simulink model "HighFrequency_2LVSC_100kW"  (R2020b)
settings: Solver=ode45  StartTime=0.0  StopTime=360  RelTol=1e-4  EnableMultiTasking=on
undefined symbols (not defined in the file): A, A_extheat, A_mp, AceH, AceL, ad0H, ad0L, ad1H, ad1L, ad2H, ad2L, AfH, AfL, at0H, at0L, at1H, at1L, at2H, at2L, C_V_ref, Cha1, CjcD, CjcT, Converters, Cp_Cu, Cp_wall, filter, FILTER_INT, fs, Grid_V, IGBT_len, IGBT_wid, Iq_init, J, k_box, k_mp, k_tp, kI_speed, kP_speed, L_equi, L_f1, Len_mp, Ls, nSpp, omega_m_init, omega_s, p, phi_pm, R1_cauer, R1D_bp, R2_cauer, R_f1, R_jc1, R_jc2, R_jc3, R_jc4, R_wall, Radius, RceH, RceL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
libraries: simulink x5, powerlib_meascontrol x2, pid_lib x2, cstblocks x1
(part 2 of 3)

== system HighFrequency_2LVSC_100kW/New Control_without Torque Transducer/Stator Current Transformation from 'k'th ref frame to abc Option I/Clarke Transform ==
  in_1 : Inport
  in_2 : Inport  Port=2
  1/w2 : Constant  Value=1/sqrt(2)
  1/w6 : Constant  Value=1/sqrt(6)
  Product : Product  InputSameDT=on  RndMeth=Zero  SaturateOnIntegerOverflow=on
  Product1 : Product  InputSameDT=on  RndMeth=Zero  SaturateOnIntegerOverflow=on
  Product2 : Product  InputSameDT=on  RndMeth=Zero  SaturateOnIntegerOverflow=on
  Sum : Sum  Inputs=-+  InputSameDT=on  SaturateOnIntegerOverflow=on
  Sum1 : Sum  Inputs=--  InputSameDT=on  SaturateOnIntegerOverflow=on
  w2/w3 : Constant  Value=sqrt(2/3)
  out_1 : Outport  VectorParamsAs1DForOutWhenUnconnected=off
  out_2 : Outport  Port=2  VectorParamsAs1DForOutWhenUnconnected=off
  out_3 : Outport  Port=3  VectorParamsAs1DForOutWhenUnconnected=off
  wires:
  in_1/1 -> Product/2, Product1/1
  Product2/1 -> Sum1/2, Sum/2
  Product1/1 -> Sum1/1, Sum/1
  1/w2/1 -> Product2/2
  1/w6/1 -> Product1/2
  w2/w3/1 -> Product/1
  Product/1 -> out_1/1
  Sum/1 -> out_2/1
  in_2/1 -> Product2/1
  Sum1/1 -> out_3/1

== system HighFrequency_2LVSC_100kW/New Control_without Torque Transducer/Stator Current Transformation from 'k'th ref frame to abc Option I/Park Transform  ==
  in_1 : Inport
  in_2 : Inport  Port=2
  in_3 : Inport  Port=3
  Product{,1..3} (4 alike) : Product  InputSameDT=on  RndMeth=Zero  SaturateOnIntegerOverflow=on
  Sum : Sum  Inputs=+-  InputSameDT=on  SaturateOnIntegerOverflow=on
  Sum1 : Sum  InputSameDT=on  SaturateOnIntegerOverflow=on
  cos : Fcn  Expr=cos(u(1))
  sin : Fcn  Expr=sin(u(1))
  out_1 : Outport  VectorParamsAs1DForOutWhenUnconnected=off
  out_2 : Outport  Port=2  VectorParamsAs1DForOutWhenUnconnected=off
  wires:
  Product2/1 -> Sum/2
  Product3/1 -> Sum1/1
  Product1/1 -> Sum/1
  Product/1 -> Sum1/2
  in_3/1 -> sin/1, cos/1
  sin/1 -> Product3/2, Product2/2
  cos/1 -> Product/2, Product1/2
  Sum/1 -> out_1/1
  Sum1/1 -> out_2/1
  in_1/1 -> Product3/1, Product1/1
  in_2/1 -> Product/1, Product2/1

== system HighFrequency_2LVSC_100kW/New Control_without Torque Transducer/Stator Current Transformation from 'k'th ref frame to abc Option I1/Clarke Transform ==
  in_1 : Inport
  in_2 : Inport  Port=2
  1/w2 : Constant  Value=1/sqrt(2)
  1/w6 : Constant  Value=1/sqrt(6)
  Product : Product  InputSameDT=on  RndMeth=Zero  SaturateOnIntegerOverflow=on
  Product1 : Product  InputSameDT=on  RndMeth=Zero  SaturateOnIntegerOverflow=on
  Product2 : Product  InputSameDT=on  RndMeth=Zero  SaturateOnIntegerOverflow=on
  Sum : Sum  Inputs=-+  InputSameDT=on  SaturateOnIntegerOverflow=on
  Sum1 : Sum  Inputs=--  InputSameDT=on  SaturateOnIntegerOverflow=on
  w2/w3 : Constant  Value=sqrt(2/3)
  out_1 : Outport  VectorParamsAs1DForOutWhenUnconnected=off
  out_2 : Outport  Port=2  VectorParamsAs1DForOutWhenUnconnected=off
  out_3 : Outport  Port=3  VectorParamsAs1DForOutWhenUnconnected=off
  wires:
  Sum1/1 -> out_3/1
  in_2/1 -> Product2/1
  Sum/1 -> out_2/1
  Product/1 -> out_1/1
  w2/w3/1 -> Product/1
  1/w6/1 -> Product1/2
  1/w2/1 -> Product2/2
  Product1/1 -> Sum/1, Sum1/1
  Product2/1 -> Sum/2, Sum1/2
  in_1/1 -> Product1/1, Product/2

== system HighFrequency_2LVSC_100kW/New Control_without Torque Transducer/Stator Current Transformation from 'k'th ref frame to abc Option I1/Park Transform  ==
  in_1 : Inport
  in_2 : Inport  Port=2
  in_3 : Inport  Port=3
  Product{,1..3} (4 alike) : Product  InputSameDT=on  RndMeth=Zero  SaturateOnIntegerOverflow=on
  Sum : Sum  Inputs=+-  InputSameDT=on  SaturateOnIntegerOverflow=on
  Sum1 : Sum  InputSameDT=on  SaturateOnIntegerOverflow=on
  cos : Fcn  Expr=cos(u(1))
  sin : Fcn  Expr=sin(u(1))
  out_1 : Outport  VectorParamsAs1DForOutWhenUnconnected=off
  out_2 : Outport  Port=2  VectorParamsAs1DForOutWhenUnconnected=off
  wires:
  in_2/1 -> Product2/1, Product/1
  in_1/1 -> Product1/1, Product3/1
  Sum1/1 -> out_2/1
  Sum/1 -> out_1/1
  cos/1 -> Product1/2, Product/2
  sin/1 -> Product2/2, Product3/2
  in_3/1 -> cos/1, sin/1
  Product/1 -> Sum1/2
  Product1/1 -> Sum/1
  Product3/1 -> Sum1/1
  Product2/1 -> Sum/2

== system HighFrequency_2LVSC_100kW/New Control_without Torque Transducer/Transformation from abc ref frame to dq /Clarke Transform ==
  note: u_b
  note: u_c
  note: u_a
  note: u_alpha
  note: u_beta
  in_1 : Inport
  in_2 : Inport  Port=2
  in_3 : Inport  Port=3
  1/w2 : Constant  Value=1/sqrt(2)
  1/w6 : Constant  Value=1/sqrt(6)
  Product{,1..3} (4 alike) : Product  InputSameDT=on  RndMeth=Zero  SaturateOnIntegerOverflow=on
  Sum : Sum  Inputs=+--  InputSameDT=on  SaturateOnIntegerOverflow=on
  Sum1 : Sum  Inputs=+-  InputSameDT=on  SaturateOnIntegerOverflow=on
  w2/w3 : Constant  Value=sqrt(2/3)
  out_1 : Outport  VectorParamsAs1DForOutWhenUnconnected=off
  out_2 : Outport  Port=2  VectorParamsAs1DForOutWhenUnconnected=off
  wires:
  Product3/1 -> out_2/1
  Sum/1 -> out_1/1
  in_1/1 -> Product/2
  Product/1 -> Sum/1
  w2/w3/1 -> Product/1
  1/w6/1 -> Product1/2, Product2/2
  Product1/1 -> Sum/2
  in_2/1 -> Sum1/1, Product1/1
  in_3/1 -> Sum1/2, Product2/1
  Sum1/1 -> Product3/1
  Product2/1 -> Sum/3
  1/w2/1 -> Product3/2

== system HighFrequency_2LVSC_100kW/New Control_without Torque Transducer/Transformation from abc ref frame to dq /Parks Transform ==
  in_1 : Inport
  in_2 : Inport  Port=2
  in_3 : Inport  Port=3
  Product{,1..3} (4 alike) : Product  InputSameDT=on  RndMeth=Zero  SaturateOnIntegerOverflow=on
  Sum : Sum  Inputs=+-  InputSameDT=on  SaturateOnIntegerOverflow=on
  Sum1 : Sum  InputSameDT=on  SaturateOnIntegerOverflow=on
  cos : Fcn  Expr=cos(u(1))
  sin : Fcn  Expr=sin(u(1))
  out_1 : Outport  VectorParamsAs1DForOutWhenUnconnected=off
  out_2 : Outport  Port=2  VectorParamsAs1DForOutWhenUnconnected=off
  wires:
  Product2/1 -> Sum/2
  Product3/1 -> Sum1/1
  Product1/1 -> Sum/1
  Product/1 -> Sum1/2
  in_3/1 -> sin/1, cos/1
  sin/1 -> Product3/2, Product2/2
  cos/1 -> Product/2, Product1/2
  Sum/1 -> out_1/1
  Sum1/1 -> out_2/1
  in_1/1 -> Product3/1, Product1/1
  in_2/1 -> Product/1, Product2/1

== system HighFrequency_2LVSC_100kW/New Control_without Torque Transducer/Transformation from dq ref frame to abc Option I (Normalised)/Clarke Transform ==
  in_1 : Inport
  in_2 : Inport  Port=2
  1/w2 : Constant  Value=1/sqrt(2)
  1/w6 : Constant  Value=1/sqrt(6)
  Product : Product  InputSameDT=on  RndMeth=Zero  SaturateOnIntegerOverflow=on
  Product1 : Product  InputSameDT=on  RndMeth=Zero  SaturateOnIntegerOverflow=on
  Product2 : Product  InputSameDT=on  RndMeth=Zero  SaturateOnIntegerOverflow=on
  Sum : Sum  Inputs=-+  InputSameDT=on  SaturateOnIntegerOverflow=on
  Sum1 : Sum  Inputs=--  InputSameDT=on  SaturateOnIntegerOverflow=on
  w2/w3 : Constant  Value=sqrt(2/3)
  out_1 : Outport  VectorParamsAs1DForOutWhenUnconnected=off
  out_2 : Outport  Port=2  VectorParamsAs1DForOutWhenUnconnected=off
  out_3 : Outport  Port=3  VectorParamsAs1DForOutWhenUnconnected=off
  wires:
  in_1/1 -> Product/2, Product1/1
  Product2/1 -> Sum1/2, Sum/2
  Product1/1 -> Sum1/1, Sum/1
  1/w2/1 -> Product2/2
  1/w6/1 -> Product1/2
  w2/w3/1 -> Product/1
  Product/1 -> out_1/1
  Sum/1 -> out_2/1
  in_2/1 -> Product2/1
  Sum1/1 -> out_3/1

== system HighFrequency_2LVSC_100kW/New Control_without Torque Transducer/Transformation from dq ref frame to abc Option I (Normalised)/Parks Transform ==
  in_1 : Inport
  in_2 : Inport  Port=2
  in_3 : Inport  Port=3
  Product{,1..3} (4 alike) : Product  InputSameDT=on  RndMeth=Zero  SaturateOnIntegerOverflow=on
  Sum : Sum  Inputs=+-  InputSameDT=on  SaturateOnIntegerOverflow=on
  Sum1 : Sum  InputSameDT=on  SaturateOnIntegerOverflow=on
  cos : Fcn  Expr=cos(u(1))
  sin : Fcn  Expr=sin(u(1))
  out_1 : Outport  VectorParamsAs1DForOutWhenUnconnected=off
  out_2 : Outport  Port=2  VectorParamsAs1DForOutWhenUnconnected=off
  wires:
  Product2/1 -> Sum/2
  Product3/1 -> Sum1/1
  Product1/1 -> Sum/1
  Product/1 -> Sum1/2
  in_3/1 -> sin/1, cos/1
  sin/1 -> Product3/2, Product2/2
  cos/1 -> Product/2, Product1/2
  Sum/1 -> out_1/1
  Sum1/1 -> out_2/1
  in_1/1 -> Product3/1, Product1/1
  in_2/1 -> Product/1, Product2/1

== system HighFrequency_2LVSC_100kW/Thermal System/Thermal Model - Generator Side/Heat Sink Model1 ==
  PT1/D1 : Inport
  Flow Rate : Inport  Port=2
  MATLAB Function : MATLAB Function  TreatAsAtomicUnit=on
  Thermal Capacitance : Constant  Value=5.8824e+03
  "Thermal System " : Subsystem
  Tha1 : Outport  VectorParamsAs1DForOutWhenUnconnected=off
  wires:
  "Thermal System "/1(Tha) -> Tha1/1
  MATLAB Function/1(y) -> "Thermal System "/2(1/R_th)  "1/R_th"
  Flow Rate/1 -> MATLAB Function/1(u)
  PT1/D1/1 -> "Thermal System "/1(P1/D1)
  Thermal Capacitance/1 -> "Thermal System "/3(C)

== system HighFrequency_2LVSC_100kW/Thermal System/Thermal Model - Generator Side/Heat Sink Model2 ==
  PT1/D1 : Inport
  Flow Rate : Inport  Port=2
  1/Rha1 : Constant  Value=1/Rha1
  MATLAB Function : MATLAB Function  Commented=on  TreatAsAtomicUnit=on
  Thermal Capacitance : Constant  Commented=on  Value=5.8824e+03
  Thermal Capacitance1 : Constant  Value=Cha1
  "Thermal System " : Subsystem
  Tha1 : Outport  VectorParamsAs1DForOutWhenUnconnected=off
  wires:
  "Thermal System "/1(Tha) -> Tha1/1
  Flow Rate/1 -> MATLAB Function/1(u)
  PT1/D1/1 -> "Thermal System "/1(P1/D1)
  Thermal Capacitance1/1 -> "Thermal System "/3(C)
  1/Rha1/1 -> "Thermal System "/2(1/R_th)

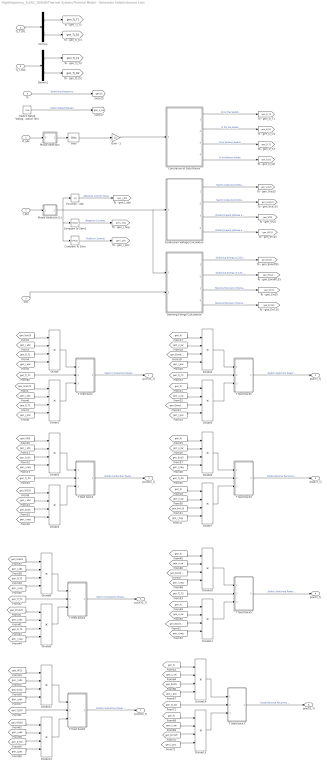
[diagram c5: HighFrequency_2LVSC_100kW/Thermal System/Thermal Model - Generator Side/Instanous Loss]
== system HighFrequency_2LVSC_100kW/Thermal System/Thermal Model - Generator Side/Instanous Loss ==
  D_abc : Inport
  I_abc : Inport  Port=2
  Vdc : Inport  Port=3
  fs : Inport  Port=4
  Tj_T1D1 : Inport  Port=5
  Tj_T2D2 : Inport  Port=6
  Bias : Bias  Bias=1
  Calculation of Duty Ratios : Subsystem
  Compare To Zero : simulink/Logic and Bit Operations/Compare To Zero  relop=>=  OutDataTypeStr=boolean
  Compare To Zero1 : simulink/Logic and Bit Operations/Compare To Zero  relop=<  OutDataTypeStr=boolean
  Conduction Voltage Calculation : Subsystem
  Demux : Demux  Outputs=2
  Demux1 : Demux  Outputs=2
  Divide{,1..15} (16 alike) : Product  Inputs=****
  Function - abs : Abs
  Gain - 1 : Gain  Gain=1/2
  Phase Selection : Subsystem
  Phase Selection (1) : Subsystem
  Switch Rated Voltage (from Initialisation file) : Constant  Value=Usw
  Swithing Energy Calculation : Subsystem
  T feed back : Subsystem
  T feed back1 : Subsystem
  T feed back2 : Subsystem
  T feed back3 : Subsystem
  T feed back4 : Subsystem
  T feed back5 : Subsystem
  T feed back6 : Subsystem
  T feed back7 : Subsystem
  pconT1_Tj : Outport  VectorParamsAs1DForOutWhenUnconnected=off
  pswT1_Tj : Outport  Port=2  VectorParamsAs1DForOutWhenUnconnected=off
  pconD1_Tj : Outport  Port=3  VectorParamsAs1DForOutWhenUnconnected=off
  pswD1_Tj : Outport  Port=4  VectorParamsAs1DForOutWhenUnconnected=off
  pconT2_Tj : Outport  Port=5  VectorParamsAs1DForOutWhenUnconnected=off
  pswT2_Tj : Outport  Port=6  VectorParamsAs1DForOutWhenUnconnected=off
  pconD2_Tj : Outport  Port=7  VectorParamsAs1DForOutWhenUnconnected=off
  pswD2_Tj : Outport  Port=8  VectorParamsAs1DForOutWhenUnconnected=off
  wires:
  D_abc/1 -> Phase Selection/1(In)
  Calculation of Duty Ratios/1(D_T1) -> [gen_D_T1]  "D for Top Switch"
  Calculation of Duty Ratios/2(D_D1) -> [gen_D_D1]  "D for Top Diode"
  Calculation of Duty Ratios/3(D_T2) -> [gen_D_T2]  "D for Bottom Switch"
  Calculation of Duty Ratios/4(D_D2) -> [gen_D_D2]  "D for Bottom Diode"
  Conduction Voltage Calculation/2(Vce 125) -> [gen_Vce125]  "Switch Collector-Emitter Voltage at 125degC"
  Conduction Voltage Calculation/4(Vf 125) -> [gen_Vf125]  "Diode Forward Voltage at 125degC"
  Conduction Voltage Calculation/1(Vce 25) -> [gen_Vce25]  "Switch Collector-Emitter Voltage at 25degC"
  Conduction Voltage Calculation/3(Vf 25) -> [gen_Vf25]  "Diode Forward Voltage at 25degC"
  Swithing Energy Calculation/4(Err 125) -> [gen_Err125]  "Reverse Recovery Energy at 125degC"
  Swithing Energy Calculation/2(Esw 125) -> [gen_Eonoff125]  "Switching Energy at 125degC"
  Swithing Energy Calculation/3(Err 25) -> [gen_Err25]  "Reverse Recovery Energy at 25degC"
  Swithing Energy Calculation/1(Esw 25) -> [gen_Eonoff25]  "Switching Energy at 25degC"
  Compare To Zero1/1 -> [gen_i_neg]  "Negative Currents"
  Compare To Zero/1 -> [gen_i_pos]  "Positive Currents"
  fs/1 -> [gen_fs]  "Switching Frequency"
  [gen_i_abs] -> Divide/2
  [gen_D_T1] -> Divide/3
  [gen_i_pos] -> Divide/4
  Function - abs/1 -> [gen_i_abs]  "Absolute Current Value"
  [gen_Vce125] -> Divide1/1
  [gen_i_abs] -> Divide1/2
  [gen_D_T1] -> Divide1/3
  [gen_i_pos] -> Divide1/4
  [gen_Vce25] -> Divide/1
  [gen_i_abs] -> Divide2/2
  [gen_D_D1] -> Divide2/3
  [gen_i_neg] -> Divide2/4
  [gen_Vf125] -> Divide3/1
  [gen_i_abs] -> Divide3/2
  [gen_D_D1] -> Divide3/3
  [gen_i_neg] -> Divide3/4
  [gen_Vf25] -> Divide2/1
  [gen_fs] -> Divide4/1
  [gen_u_sw] -> Divide4/2
  Switch Rated Voltage (from Initialisation file)/1 -> [gen_u_sw]  "Switch Rated Voltage"
  [gen_Eonoff25] -> Divide4/3
  [gen_i_pos] -> Divide4/4
  [gen_fs] -> Divide5/1
  [gen_u_sw] -> Divide5/2
  [gen_Eonoff125] -> Divide5/3
  [gen_i_pos] -> Divide5/4
  [gen_fs] -> Divide6/1
  [gen_u_sw] -> Divide6/2
  [gen_Err25] -> Divide6/3
  [gen_i_neg] -> Divide6/4
  [gen_fs] -> Divide7/1
  [gen_u_sw] -> Divide7/2
  [gen_Err125] -> Divide7/3
  [gen_i_neg] -> Divide7/4
  Divide4/1 -> T feed back1/1(TL)
  Divide5/1 -> T feed back1/3(TH)
  Divide/1 -> T feed back/1(TL)
  Divide1/1 -> T feed back/3(TH)
  T feed back/1(p_Tj) -> pconT1_Tj/1  "Switch Conduction Power Loss at Tj"
  Tj_T1D1/1 -> Demux/1
  Demux/1 -> [gen_Tj_T1]
  Demux/2 -> [gen_Tj_D1]
  [gen_Tj_T1] -> T feed back/2(Tj)
  [gen_Tj_T1] -> T feed back1/2(Tj)
  T feed back1/1(p_Tj) -> pswT1_Tj/1  "Switch Switching Power Loss at Tj"
  Divide2/1 -> T feed back2/1(TL)
  Divide3/1 -> T feed back2/3(TH)
  [gen_Tj_D1] -> T feed back2/2(Tj)
  T feed back2/1(p_Tj) -> pconD1_Tj/1  "Diode Conduction Power Loss at Tj"
  [gen_Tj_D1] -> T feed back3/2(Tj)
  Divide6/1 -> T feed back3/1(TL)
  Divide7/1 -> T feed back3/3(TH)
  T feed back3/1(p_Tj) -> pswD1_Tj/1  "Diode Reverse Recovery Power Loss at Tj"
  I_abc/1 -> Phase Selection (1)/1(In)
  Vdc/1 -> Swithing Energy Calculation/2(Vdc)
  Phase Selection (1)/1(Out) -> Swithing Energy Calculation/1(i_abc), Conduction Voltage Calculation/1(i_abc), Compare To Zero/1, Compare To Zero1/1, Function - abs/1
  Bias/1 -> Gain - 1/1
  Phase Selection/1(Out) -> Bias/1
  Gain - 1/1 -> Calculation of Duty Ratios/1(Dabc)
  Tj_T2D2/1 -> Demux1/1
  Demux1/1 -> [gen_Tj_T2]
  Demux1/2 -> [gen_Tj_D2]
  [gen_i_abs] -> Divide8/2
  [gen_D_T2] -> Divide8/3
  [gen_i_neg] -> Divide8/4
  [gen_Vce125] -> Divide9/1
  [gen_i_abs] -> Divide9/2
  [gen_D_T2] -> Divide9/3
  [gen_i_neg] -> Divide9/4
  [gen_Vce25] -> Divide8/1
  Divide8/1 -> T feed back4/1(TL)
  Divide9/1 -> T feed back4/3(TH)
  T feed back4/1(p_Tj) -> pconT2_Tj/1  "Switch Conduction Power Loss at Tj"
  [gen_Tj_T2] -> T feed back4/2(Tj)
  [gen_fs] -> Divide10/1
  [gen_u_sw] -> Divide10/2
  [gen_Eonoff25] -> Divide10/3
  [gen_i_neg] -> Divide10/4
  [gen_fs] -> Divide11/1
  [gen_u_sw] -> Divide11/2
  [gen_Eonoff125] -> Divide11/3
  [gen_i_neg] -> Divide11/4
  Divide10/1 -> T feed back5/1(TL)
  Divide11/1 -> T feed back5/3(TH)
  [gen_Tj_T2] -> T feed back5/2(Tj)
  T feed back5/1(p_Tj) -> pswT2_Tj/1  "Switch Switching Power Loss at Tj"
  [gen_i_abs] -> Divide12/2
  [gen_D_D2] -> Divide12/3
  [gen_i_pos] -> Divide12/4
  [gen_Vf125] -> Divide13/1
  [gen_i_abs] -> Divide13/2
  [gen_D_D2] -> Divide13/3
  [gen_i_pos] -> Divide13/4
  [gen_Vf25] -> Divide12/1
  Divide12/1 -> T feed back6/1(TL)
  Divide13/1 -> T feed back6/3(TH)
  [gen_Tj_D2] -> T feed back6/2(Tj)
  T feed back6/1(p_Tj) -> pconD2_Tj/1  "Diode Conduction Power Loss at Tj"
  [gen_fs] -> Divide14/1
  [gen_u_sw] -> Divide14/2
  [gen_Err25] -> Divide14/3
  [gen_i_pos] -> Divide14/4
  [gen_fs] -> Divide15/1
  [gen_u_sw] -> Divide15/2
  [gen_Err125] -> Divide15/3
  [gen_i_pos] -> Divide15/4
  [gen_Tj_D2] -> T feed back7/2(Tj)
  Divide14/1 -> T feed back7/1(TL)
  Divide15/1 -> T feed back7/3(TH)
  T feed back7/1(p_Tj) -> pswD2_Tj/1  "Diode Reverse Recovery Power Loss at Tj"

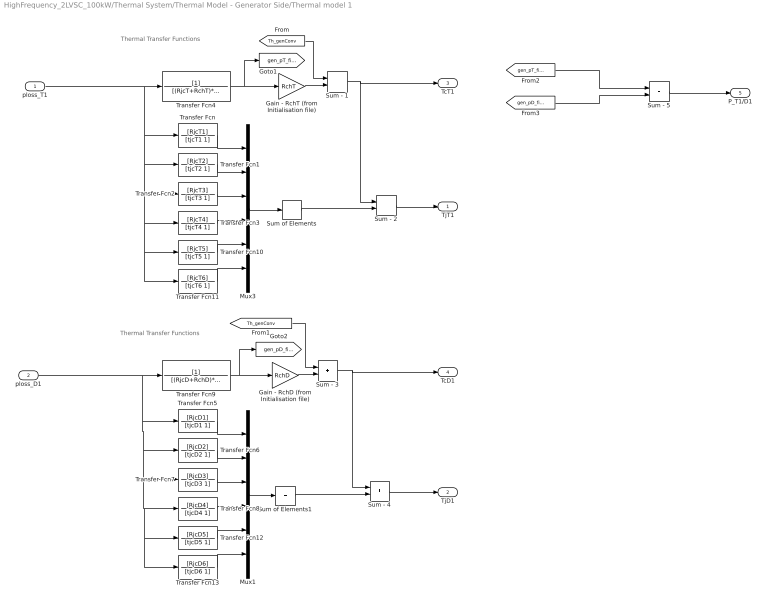
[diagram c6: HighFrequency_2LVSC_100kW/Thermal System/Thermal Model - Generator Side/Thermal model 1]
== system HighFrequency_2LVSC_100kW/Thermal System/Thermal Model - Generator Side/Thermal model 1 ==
  note: Thermal Transfer Functions
  note: Thermal Transfer Functions
  ploss_T1 : Inport
  ploss_D1 : Inport  Port=2
  Gain - RchD (from Initialisation file) : Gain  Gain=RchD
  Gain - RchT (from Initialisation file) : Gain  Gain=RchT
  Mux1 : Mux  Inputs=6
  Mux3 : Mux  Inputs=6
  Sum - {1..5} (5 alike) : Sum
  Sum of Elements : Sum  Inputs=+
  Sum of Elements1 : Sum  Inputs=+
  Transfer Fcn : TransferFcn  Numerator=[RjcT1]  Denominator=[tjcT1 1]
  Transfer Fcn1 : TransferFcn  Numerator=[RjcT2]  Denominator=[tjcT2 1]
  Transfer Fcn10 : TransferFcn  Numerator=[RjcT5]  Denominator=[tjcT5 1]
  Transfer Fcn11 : TransferFcn  Numerator=[RjcT6]  Denominator=[tjcT6 1]
  Transfer Fcn12 : TransferFcn  Numerator=[RjcD5]  Denominator=[tjcD5 1]
  Transfer Fcn13 : TransferFcn  Numerator=[RjcD6]  Denominator=[tjcD6 1]
  Transfer Fcn2 : TransferFcn  Numerator=[RjcT3]  Denominator=[tjcT3 1]
  Transfer Fcn3 : TransferFcn  Numerator=[RjcT4]  Denominator=[tjcT4 1]
  Transfer Fcn4 : TransferFcn  Denominator=[(RjcT+RchT)*CjcT 1]
  Transfer Fcn5 : TransferFcn  Numerator=[RjcD1]  Denominator=[tjcD1 1]
  Transfer Fcn6 : TransferFcn  Numerator=[RjcD2]  Denominator=[tjcD2 1]
  Transfer Fcn7 : TransferFcn  Numerator=[RjcD3]  Denominator=[tjcD3 1]
  Transfer Fcn8 : TransferFcn  Numerator=[RjcD4]  Denominator=[tjcD4 1]
  Transfer Fcn9 : TransferFcn  Denominator=[(RjcD+RchD)*CjcD 1]
  TjT1 : Outport  VectorParamsAs1DForOutWhenUnconnected=off
  TjD1 : Outport  Port=2  VectorParamsAs1DForOutWhenUnconnected=off
  TcT1 : Outport  Port=3  VectorParamsAs1DForOutWhenUnconnected=off
  TcD1 : Outport  Port=4  VectorParamsAs1DForOutWhenUnconnected=off
  P_T1/D1 : Outport  Port=5  VectorParamsAs1DForOutWhenUnconnected=off
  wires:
  Mux3/1 -> Sum of Elements/1
  Transfer Fcn3/1 -> Mux3/4
  Transfer Fcn1/1 -> Mux3/2
  Transfer Fcn2/1 -> Mux3/3
  Transfer Fcn/1 -> Mux3/1
  Mux1/1 -> Sum of Elements1/1
  Sum of Elements1/1 -> Sum - 4/2
  Transfer Fcn8/1 -> Mux1/4
  Transfer Fcn6/1 -> Mux1/2
  Transfer Fcn7/1 -> Mux1/3
  Transfer Fcn5/1 -> Mux1/1
  Transfer Fcn4/1 -> [gen_pT_filter], Gain - RchT (from Initialisation file)/1
  Transfer Fcn9/1 -> [gen_pD_filter], Gain - RchD (from Initialisation file)/1
  ploss_D1/1 -> Transfer Fcn9/1, Transfer Fcn5/1, Transfer Fcn13/1, Transfer Fcn12/1, Transfer Fcn8/1, Transfer Fcn7/1, Transfer Fcn6/1
  Gain - RchT (from Initialisation file)/1 -> Sum - 1/2
  Sum of Elements/1 -> Sum - 2/2
  Sum - 1/1 -> Sum - 2/1, TcT1/1
  Sum - 2/1 -> TjT1/1
  Sum - 4/1 -> TjD1/1
  Sum - 3/1 -> Sum - 4/1, TcD1/1
  Gain - RchD (from Initialisation file)/1 -> Sum - 3/2
  Transfer Fcn10/1 -> Mux3/5
  Transfer Fcn11/1 -> Mux3/6
  Transfer Fcn12/1 -> Mux1/5
  Transfer Fcn13/1 -> Mux1/6
  [gen_pT_filter] -> Sum - 5/1
  [gen_pD_filter] -> Sum - 5/2
  Sum - 5/1 -> P_T1/D1/1
  [Th_genConv] -> Sum - 1/1
  [Th_genConv] -> Sum - 3/1
  ploss_T1/1 -> Transfer Fcn4/1, Transfer Fcn11/1, Transfer Fcn10/1, Transfer Fcn3/1, Transfer Fcn2/1, Transfer Fcn1/1, Transfer Fcn/1

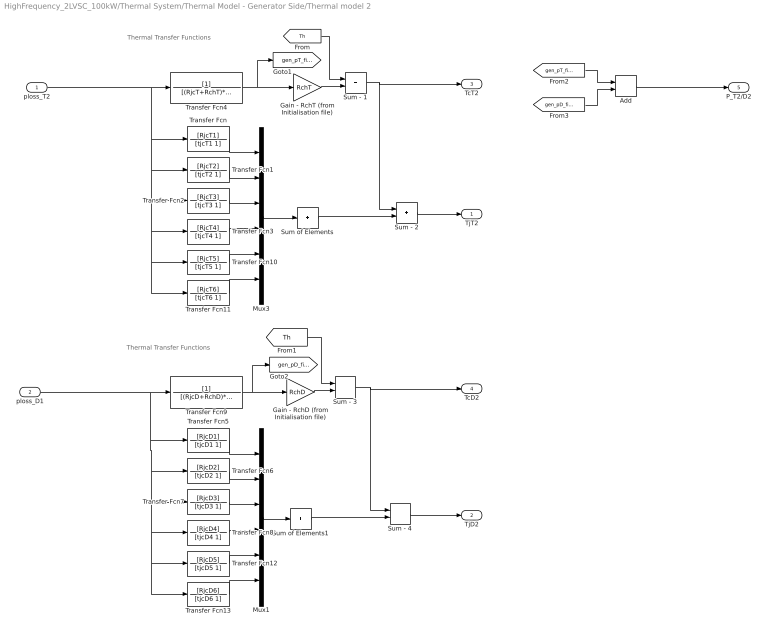
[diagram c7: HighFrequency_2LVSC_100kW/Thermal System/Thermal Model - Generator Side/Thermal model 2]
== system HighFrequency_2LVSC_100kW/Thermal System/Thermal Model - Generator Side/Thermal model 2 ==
  note: Thermal Transfer Functions
  note: Thermal Transfer Functions
  ploss_T2 : Inport
  ploss_D1 : Inport  Port=2
  Add : Sum
  Gain - RchD (from Initialisation file) : Gain  Gain=RchD
  Gain - RchT (from Initialisation file) : Gain  Gain=RchT
  Mux1 : Mux  Inputs=6
  Mux3 : Mux  Inputs=6
  Sum - {1..4} (4 alike) : Sum
  Sum of Elements : Sum  Inputs=+
  Sum of Elements1 : Sum  Inputs=+
  Transfer Fcn : TransferFcn  Numerator=[RjcT1]  Denominator=[tjcT1 1]
  Transfer Fcn1 : TransferFcn  Numerator=[RjcT2]  Denominator=[tjcT2 1]
  Transfer Fcn10 : TransferFcn  Numerator=[RjcT5]  Denominator=[tjcT5 1]
  Transfer Fcn11 : TransferFcn  Numerator=[RjcT6]  Denominator=[tjcT6 1]
  Transfer Fcn12 : TransferFcn  Numerator=[RjcD5]  Denominator=[tjcD5 1]
  Transfer Fcn13 : TransferFcn  Numerator=[RjcD6]  Denominator=[tjcD6 1]
  Transfer Fcn2 : TransferFcn  Numerator=[RjcT3]  Denominator=[tjcT3 1]
  Transfer Fcn3 : TransferFcn  Numerator=[RjcT4]  Denominator=[tjcT4 1]
  Transfer Fcn4 : TransferFcn  Denominator=[(RjcT+RchT)*CjcT 1]
  Transfer Fcn5 : TransferFcn  Numerator=[RjcD1]  Denominator=[tjcD1 1]
  Transfer Fcn6 : TransferFcn  Numerator=[RjcD2]  Denominator=[tjcD2 1]
  Transfer Fcn7 : TransferFcn  Numerator=[RjcD3]  Denominator=[tjcD3 1]
  Transfer Fcn8 : TransferFcn  Numerator=[RjcD4]  Denominator=[tjcD4 1]
  Transfer Fcn9 : TransferFcn  Denominator=[(RjcD+RchD)*CjcD 1]
  TjT2 : Outport  VectorParamsAs1DForOutWhenUnconnected=off
  TjD2 : Outport  Port=2  VectorParamsAs1DForOutWhenUnconnected=off
  TcT2 : Outport  Port=3  VectorParamsAs1DForOutWhenUnconnected=off
  TcD2 : Outport  Port=4  VectorParamsAs1DForOutWhenUnconnected=off
  P_T2/D2 : Outport  Port=5  VectorParamsAs1DForOutWhenUnconnected=off
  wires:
  Mux3/1 -> Sum of Elements/1
  Transfer Fcn3/1 -> Mux3/4
  Transfer Fcn1/1 -> Mux3/2
  Transfer Fcn2/1 -> Mux3/3
  Transfer Fcn/1 -> Mux3/1
  Mux1/1 -> Sum of Elements1/1
  Sum of Elements1/1 -> Sum - 4/2
  Transfer Fcn8/1 -> Mux1/4
  Transfer Fcn6/1 -> Mux1/2
  Transfer Fcn7/1 -> Mux1/3
  Transfer Fcn5/1 -> Mux1/1
  Transfer Fcn4/1 -> [gen_pT_filter], Gain - RchT (from Initialisation file)/1
  Transfer Fcn9/1 -> [gen_pD_filter], Gain - RchD (from Initialisation file)/1
  ploss_D1/1 -> Transfer Fcn9/1, Transfer Fcn5/1, Transfer Fcn13/1, Transfer Fcn12/1, Transfer Fcn8/1, Transfer Fcn7/1, Transfer Fcn6/1
  Gain - RchT (from Initialisation file)/1 -> Sum - 1/2
  Sum of Elements/1 -> Sum - 2/2
  Sum - 1/1 -> Sum - 2/1, TcT2/1
  Sum - 2/1 -> TjT2/1
  Sum - 4/1 -> TjD2/1
  Sum - 3/1 -> Sum - 4/1, TcD2/1
  Gain - RchD (from Initialisation file)/1 -> Sum - 3/2
  Transfer Fcn10/1 -> Mux3/5
  Transfer Fcn11/1 -> Mux3/6
  Transfer Fcn12/1 -> Mux1/5
  Transfer Fcn13/1 -> Mux1/6
  [Th] -> Sum - 1/1
  [Th] -> Sum - 3/1
  [gen_pT_filter] -> Add/1
  [gen_pD_filter] -> Add/2
  ploss_T2/1 -> Transfer Fcn4/1, Transfer Fcn11/1, Transfer Fcn10/1, Transfer Fcn3/1, Transfer Fcn2/1, Transfer Fcn1/1, Transfer Fcn/1
  Add/1 -> P_T2/D2/1

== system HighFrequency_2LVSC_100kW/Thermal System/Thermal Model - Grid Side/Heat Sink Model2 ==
  PT1/D1 : Inport
  Forced Cooling TrFn : TransferFcn  Commented=on  Numerator=[Rha1]  Denominator=[tha1 1]
  Natural Cooling 1 : Subsystem
  Tha : Outport  VectorParamsAs1DForOutWhenUnconnected=off
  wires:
  Natural Cooling 1/1(Tc_trfn) -> Tha/1
  PT1/D1/1 -> Natural Cooling 1/1(Filtered Loss)

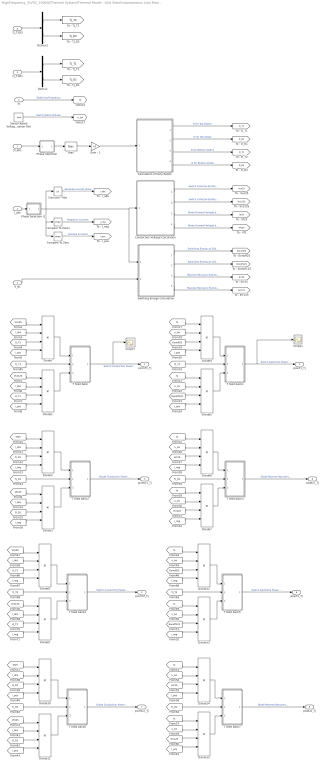
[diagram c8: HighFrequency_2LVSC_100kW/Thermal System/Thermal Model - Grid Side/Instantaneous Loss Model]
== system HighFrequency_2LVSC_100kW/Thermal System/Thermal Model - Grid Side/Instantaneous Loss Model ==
  D_abc : Inport
  I_abc : Inport  Port=2
  V_dc : Inport  Port=3
  fs : Inport  Port=4
  Tj_T1D1 : Inport  Port=5
  Tj_T2D2 : Inport  Port=6
  Bias : Bias  Bias=1
  Calculation of Duty Ratios : Subsystem
  Compare To Zero : simulink/Logic and Bit Operations/Compare To Zero  relop=>=  OutDataTypeStr=boolean
  Compare To Zero1 : simulink/Logic and Bit Operations/Compare To Zero  relop=<  OutDataTypeStr=boolean
  Conduction Voltage Calculation : Subsystem
  Demux : Demux  Outputs=2
  Demux1 : Demux  Outputs=2
  Divide{,1..15} (16 alike) : Product  Inputs=****
  Function - Abs : Abs
  Gain - 1 : Gain  Gain=1/2
  Phase Selection : Subsystem
  Phase Selection (1) : Subsystem
  Scope1 : Scope
  Scope7 : Scope
  Switch Rated Voltage (from Initialisation file) : Constant  Value=Usw
  Swithing Energy Calculation : Subsystem
  T feed back : Subsystem
  T feed back1 : Subsystem
  T feed back2 : Subsystem
  T feed back3 : Subsystem
  T feed back4 : Subsystem
  T feed back5 : Subsystem
  T feed back6 : Subsystem
  T feed back7 : Subsystem
  pconT1_Tj : Outport  VectorParamsAs1DForOutWhenUnconnected=off
  pswT1_Tj : Outport  Port=2  VectorParamsAs1DForOutWhenUnconnected=off
  pconD1_Tj : Outport  Port=3  VectorParamsAs1DForOutWhenUnconnected=off
  pswD1_Tj : Outport  Port=4  VectorParamsAs1DForOutWhenUnconnected=off
  pconT2_Tj : Outport  Port=5  VectorParamsAs1DForOutWhenUnconnected=off
  pswT2_Tj : Outport  Port=6  VectorParamsAs1DForOutWhenUnconnected=off
  pconD2_Tj : Outport  Port=7  VectorParamsAs1DForOutWhenUnconnected=off
  pswD2_Tj : Outport  Port=8  VectorParamsAs1DForOutWhenUnconnected=off
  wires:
  D_abc/1 -> Phase Selection/1(In)
  Calculation of Duty Ratios/1(D_T1) -> [D_T1]  "D for Top Switch"
  Calculation of Duty Ratios/2(D_D1) -> [D_D1]  "D for Top Diode"
  Calculation of Duty Ratios/3(D_T2) -> [D_T2]  "D for Bottom Switch"
  Calculation of Duty Ratios/4(D_D2) -> [D_D2]  "D for Bottom Diode"
  Conduction Voltage Calculation/2(Vce 125) -> [Vce125]  "Switch Collector-Emitter Voltage at 125degC"
  Conduction Voltage Calculation/4(Vf 125) -> [Vf125]  "Diode Forward Voltage at 125degC"
  Conduction Voltage Calculation/1(Vce 25) -> [Vce25]  "Switch Collector-Emitter Voltage at 25degC"
  Conduction Voltage Calculation/3(Vf 25) -> [Vf25]  "Diode Forward Voltage at 25degC"
  Swithing Energy Calculation/4(Err 125) -> [Err125]  "Reverse Recovery Energy at 125degC"
  Swithing Energy Calculation/2(Esw 125) -> [Eonoff125]  "Switching Energy at 125degC"
  Swithing Energy Calculation/3(Err 25) -> [Err25]  "Reverse Recovery Energy at 25degC"
  Swithing Energy Calculation/1(Esw 25) -> [Eonoff25]  "Switching Energy at 25degC"
  Compare To Zero1/1 -> [i_neg]  "Negative Currents"
  Compare To Zero/1 -> [i_pos]  "Positive Currents"
  fs/1 -> [fs]  "Switching Frequency"
  [i_abs] -> Divide/2
  [D_T1] -> Divide/3
  [i_pos] -> Divide/4
  Function - Abs/1 -> [i_abs]  "Absolute Current Value"
  [Vce125] -> Divide1/1
  [i_abs] -> Divide1/2
  [D_T1] -> Divide1/3
  [i_pos] -> Divide1/4
  [Vce25] -> Divide/1
  [i_abs] -> Divide2/2
  [D_D1] -> Divide2/3
  [i_neg] -> Divide2/4
  [Vf125] -> Divide3/1
  [i_abs] -> Divide3/2
  [D_D1] -> Divide3/3
  [i_neg] -> Divide3/4
  [Vf25] -> Divide2/1
  [fs] -> Divide4/1
  [u_sw] -> Divide4/2
  Switch Rated Voltage (from Initialisation file)/1 -> [u_sw]  "Switch Rated Voltage"
  [Eonoff25] -> Divide4/3
  [i_pos] -> Divide4/4
  [fs] -> Divide5/1
  [u_sw] -> Divide5/2
  [Eonoff125] -> Divide5/3
  [i_pos] -> Divide5/4
  [fs] -> Divide6/1
  [u_sw] -> Divide6/2
  [Err25] -> Divide6/3
  [i_neg] -> Divide6/4
  [fs] -> Divide7/1
  [u_sw] -> Divide7/2
  [Err125] -> Divide7/3
  [i_neg] -> Divide7/4
  Divide4/1 -> T feed back1/1(TL)
  Divide5/1 -> T feed back1/3(TH)
  Divide/1 -> T feed back/1(TL)
  Divide1/1 -> T feed back/3(TH)
  T feed back/1(p_Tj) -> Scope7/1, pconT1_Tj/1  "Switch Conduction Power Loss at Tj"
  Tj_T1D1/1 -> Demux/1
  Demux/1 -> [Tj_T1]
  Demux/2 -> [Tj_D1]
  [Tj_T1] -> T feed back/2(Tj)
  [Tj_T1] -> T feed back1/2(Tj)
  T feed back1/1(p_Tj) -> Scope1/1, pswT1_Tj/1  "Switch Switching Power Loss at Tj"
  Divide2/1 -> T feed back2/1(TL)
  Divide3/1 -> T feed back2/3(TH)
  [Tj_D1] -> T feed back2/2(Tj)
  T feed back2/1(p_Tj) -> pconD1_Tj/1  "Diode Conduction Power Loss at Tj"
  [Tj_D1] -> T feed back3/2(Tj)
  Divide6/1 -> T feed back3/1(TL)
  Divide7/1 -> T feed back3/3(TH)
  T feed back3/1(p_Tj) -> pswD1_Tj/1  "Diode Reverse Recovery Power Loss at Tj"
  I_abc/1 -> Phase Selection (1)/1(In)
  V_dc/1 -> Swithing Energy Calculation/2(Vdc)
  Phase Selection (1)/1(Out) -> Compare To Zero1/1, Compare To Zero/1, Swithing Energy Calculation/1(i_abc), Conduction Voltage Calculation/1(i_abc), Function - Abs/1
  Bias/1 -> Gain - 1/1
  Phase Selection/1(Out) -> Bias/1
  Gain - 1/1 -> Calculation of Duty Ratios/1(D_abc)
  Tj_T2D2/1 -> Demux1/1
  Demux1/1 -> [Tj_T2]
  Demux1/2 -> [Tj_D2]
  [i_abs] -> Divide8/2
  [D_T2] -> Divide8/3
  [i_neg] -> Divide8/4
  [Vce125] -> Divide9/1
  [i_abs] -> Divide9/2
  [D_T2] -> Divide9/3
  [i_neg] -> Divide9/4
  [Vce25] -> Divide8/1
  [i_abs] -> Divide10/2
  [D_D2] -> Divide10/3
  [i_pos] -> Divide10/4
  [Vf125] -> Divide11/1
  [i_abs] -> Divide11/2
  [D_D2] -> Divide11/3
  [i_pos] -> Divide11/4
  [Vf25] -> Divide10/1
  [fs] -> Divide12/1
  [u_sw] -> Divide12/2
  [Eonoff25] -> Divide12/3
  [i_neg] -> Divide12/4
  [fs] -> Divide13/1
  [u_sw] -> Divide13/2
  [Eonoff125] -> Divide13/3
  [i_neg] -> Divide13/4
  [fs] -> Divide14/1
  [u_sw] -> Divide14/2
  [Err25] -> Divide14/3
  [i_pos] -> Divide14/4
  [fs] -> Divide15/1
  [u_sw] -> Divide15/2
  [Err125] -> Divide15/3
  [i_pos] -> Divide15/4
  Divide12/1 -> T feed back5/1(TL)
  Divide13/1 -> T feed back5/3(TH)
  Divide8/1 -> T feed back4/1(TL)
  Divide9/1 -> T feed back4/3(TH)
  T feed back4/1(p_Tj) -> pconT2_Tj/1  "Switch Conduction Power Loss at Tj"
  [Tj_T2] -> T feed back4/2(Tj)
  [Tj_T2] -> T feed back5/2(Tj)
  T feed back5/1(p_Tj) -> pswT2_Tj/1  "Switch Switching Power Loss at Tj"
  Divide10/1 -> T feed back6/1(TL)
  Divide11/1 -> T feed back6/3(TH)
  [Tj_D2] -> T feed back6/2(Tj)
  T feed back6/1(p_Tj) -> pconD2_Tj/1  "Diode Conduction Power Loss at Tj"
  [Tj_D2] -> T feed back7/2(Tj)
  Divide14/1 -> T feed back7/1(TL)
  Divide15/1 -> T feed back7/3(TH)
  T feed back7/1(p_Tj) -> pswD2_Tj/1  "Diode Reverse Recovery Power Loss at Tj"

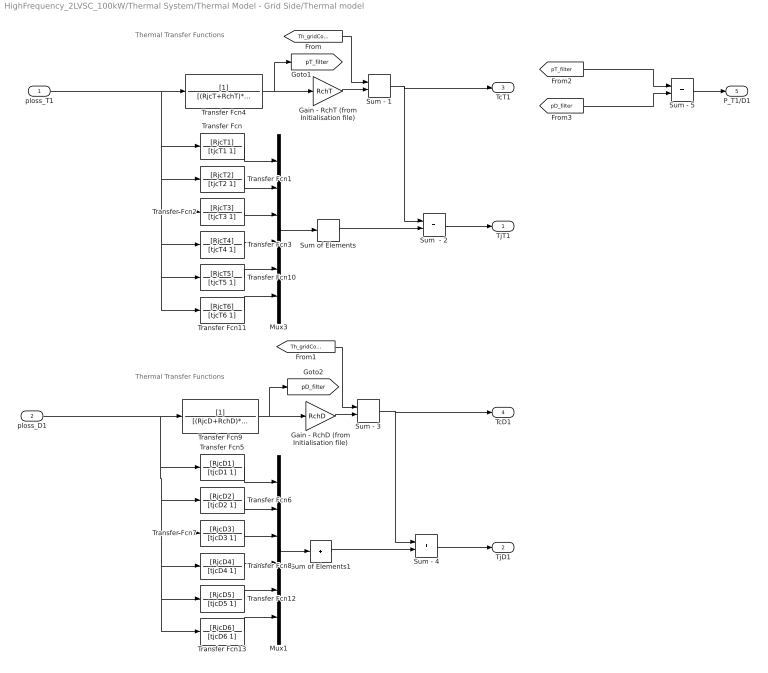
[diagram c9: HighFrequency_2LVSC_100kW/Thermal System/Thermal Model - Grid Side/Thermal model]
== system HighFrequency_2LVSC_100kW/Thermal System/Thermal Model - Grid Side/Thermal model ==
  note: Thermal Transfer Functions
  note: Thermal Transfer Functions
  ploss_T1 : Inport
  ploss_D1 : Inport  Port=2
  Gain - RchD (from Initialisation file) : Gain  Gain=RchD
  Gain - RchT (from Initialisation file) : Gain  Gain=RchT
  Mux1 : Mux  Inputs=6
  Mux3 : Mux  Inputs=6
  Sum  - 2 : Sum
  Sum - {1,3..5} (4 alike) : Sum
  Sum of Elements : Sum  Inputs=+
  Sum of Elements1 : Sum  Inputs=+
  Transfer Fcn : TransferFcn  Numerator=[RjcT1]  Denominator=[tjcT1 1]
  Transfer Fcn1 : TransferFcn  Numerator=[RjcT2]  Denominator=[tjcT2 1]
  Transfer Fcn10 : TransferFcn  Numerator=[RjcT5]  Denominator=[tjcT5 1]
  Transfer Fcn11 : TransferFcn  Numerator=[RjcT6]  Denominator=[tjcT6 1]
  Transfer Fcn12 : TransferFcn  Numerator=[RjcD5]  Denominator=[tjcD5 1]
  Transfer Fcn13 : TransferFcn  Numerator=[RjcD6]  Denominator=[tjcD6 1]
  Transfer Fcn2 : TransferFcn  Numerator=[RjcT3]  Denominator=[tjcT3 1]
  Transfer Fcn3 : TransferFcn  Numerator=[RjcT4]  Denominator=[tjcT4 1]
  Transfer Fcn4 : TransferFcn  Denominator=[(RjcT+RchT)*CjcT 1]
  Transfer Fcn5 : TransferFcn  Numerator=[RjcD1]  Denominator=[tjcD1 1]
  Transfer Fcn6 : TransferFcn  Numerator=[RjcD2]  Denominator=[tjcD2 1]
  Transfer Fcn7 : TransferFcn  Numerator=[RjcD3]  Denominator=[tjcD3 1]
  Transfer Fcn8 : TransferFcn  Numerator=[RjcD4]  Denominator=[tjcD4 1]
  Transfer Fcn9 : TransferFcn  Denominator=[(RjcD+RchD)*CjcD 1]
  TjT1 : Outport  VectorParamsAs1DForOutWhenUnconnected=off
  TjD1 : Outport  Port=2  VectorParamsAs1DForOutWhenUnconnected=off
  TcT1 : Outport  Port=3  VectorParamsAs1DForOutWhenUnconnected=off
  TcD1 : Outport  Port=4  VectorParamsAs1DForOutWhenUnconnected=off
  P_T1/D1 : Outport  Port=5  VectorParamsAs1DForOutWhenUnconnected=off
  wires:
  Mux3/1 -> Sum of Elements/1
  Transfer Fcn3/1 -> Mux3/4
  Transfer Fcn1/1 -> Mux3/2
  Transfer Fcn2/1 -> Mux3/3
  Transfer Fcn/1 -> Mux3/1
  Mux1/1 -> Sum of Elements1/1
  Sum of Elements1/1 -> Sum - 4/2
  Transfer Fcn8/1 -> Mux1/4
  Transfer Fcn6/1 -> Mux1/2
  Transfer Fcn7/1 -> Mux1/3
  Transfer Fcn5/1 -> Mux1/1
  Transfer Fcn4/1 -> [pT_filter], Gain - RchT (from Initialisation file)/1
  Transfer Fcn9/1 -> [pD_filter], Gain - RchD (from Initialisation file)/1
  ploss_D1/1 -> Transfer Fcn9/1, Transfer Fcn5/1, Transfer Fcn13/1, Transfer Fcn12/1, Transfer Fcn8/1, Transfer Fcn7/1, Transfer Fcn6/1
  Gain - RchT (from Initialisation file)/1 -> Sum - 1/2
  Sum of Elements/1 -> Sum  - 2/2
  Sum - 1/1 -> Sum  - 2/1, TcT1/1
  Sum  - 2/1 -> TjT1/1
  Sum - 4/1 -> TjD1/1
  Sum - 3/1 -> Sum - 4/1, TcD1/1
  Gain - RchD (from Initialisation file)/1 -> Sum - 3/2
  Transfer Fcn10/1 -> Mux3/5
  Transfer Fcn11/1 -> Mux3/6
  Transfer Fcn12/1 -> Mux1/5
  Transfer Fcn13/1 -> Mux1/6
  [pT_filter] -> Sum - 5/1
  Sum - 5/1 -> P_T1/D1/1
  [Th_gridConv] -> Sum - 1/1
  [pD_filter] -> Sum - 5/2
  ploss_T1/1 -> Transfer Fcn4/1, Transfer Fcn11/1, Transfer Fcn10/1, Transfer Fcn3/1, Transfer Fcn2/1, Transfer Fcn1/1, Transfer Fcn/1
  [Th_gridConv] -> Sum - 3/1

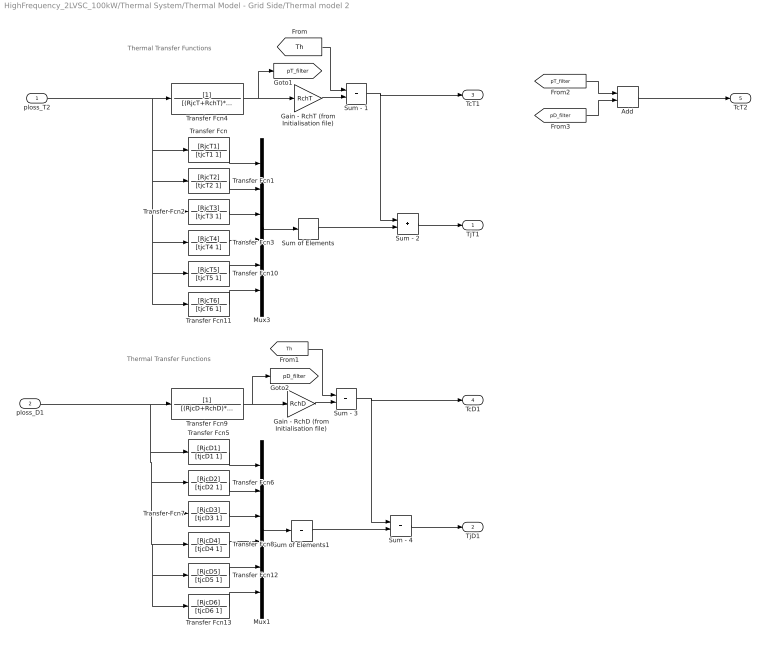
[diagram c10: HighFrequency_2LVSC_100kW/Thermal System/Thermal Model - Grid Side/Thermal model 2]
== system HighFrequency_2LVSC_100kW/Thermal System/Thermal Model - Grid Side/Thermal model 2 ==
  note: Thermal Transfer Functions
  note: Thermal Transfer Functions
  ploss_T2 : Inport
  ploss_D1 : Inport  Port=2
  Add : Sum
  Gain - RchD (from Initialisation file) : Gain  Gain=RchD
  Gain - RchT (from Initialisation file) : Gain  Gain=RchT
  Mux1 : Mux  Inputs=6
  Mux3 : Mux  Inputs=6
  Sum - {1..4} (4 alike) : Sum
  Sum of Elements : Sum  Inputs=+
  Sum of Elements1 : Sum  Inputs=+
  Transfer Fcn : TransferFcn  Numerator=[RjcT1]  Denominator=[tjcT1 1]
  Transfer Fcn1 : TransferFcn  Numerator=[RjcT2]  Denominator=[tjcT2 1]
  Transfer Fcn10 : TransferFcn  Numerator=[RjcT5]  Denominator=[tjcT5 1]
  Transfer Fcn11 : TransferFcn  Numerator=[RjcT6]  Denominator=[tjcT6 1]
  Transfer Fcn12 : TransferFcn  Numerator=[RjcD5]  Denominator=[tjcD5 1]
  Transfer Fcn13 : TransferFcn  Numerator=[RjcD6]  Denominator=[tjcD6 1]
  Transfer Fcn2 : TransferFcn  Numerator=[RjcT3]  Denominator=[tjcT3 1]
  Transfer Fcn3 : TransferFcn  Numerator=[RjcT4]  Denominator=[tjcT4 1]
  Transfer Fcn4 : TransferFcn  Denominator=[(RjcT+RchT)*CjcT 1]
  Transfer Fcn5 : TransferFcn  Numerator=[RjcD1]  Denominator=[tjcD1 1]
  Transfer Fcn6 : TransferFcn  Numerator=[RjcD2]  Denominator=[tjcD2 1]
  Transfer Fcn7 : TransferFcn  Numerator=[RjcD3]  Denominator=[tjcD3 1]
  Transfer Fcn8 : TransferFcn  Numerator=[RjcD4]  Denominator=[tjcD4 1]
  Transfer Fcn9 : TransferFcn  Denominator=[(RjcD+RchD)*CjcD 1]
  TjT1 : Outport  VectorParamsAs1DForOutWhenUnconnected=off
  TjD1 : Outport  Port=2  VectorParamsAs1DForOutWhenUnconnected=off
  TcT1 : Outport  Port=3  VectorParamsAs1DForOutWhenUnconnected=off
  TcD1 : Outport  Port=4  VectorParamsAs1DForOutWhenUnconnected=off
  TcT2 : Outport  Port=5  VectorParamsAs1DForOutWhenUnconnected=off
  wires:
  Mux3/1 -> Sum of Elements/1
  Transfer Fcn3/1 -> Mux3/4
  Transfer Fcn1/1 -> Mux3/2
  Transfer Fcn2/1 -> Mux3/3
  Transfer Fcn/1 -> Mux3/1
  Mux1/1 -> Sum of Elements1/1
  Sum of Elements1/1 -> Sum - 4/2
  Transfer Fcn8/1 -> Mux1/4
  Transfer Fcn6/1 -> Mux1/2
  Transfer Fcn7/1 -> Mux1/3
  Transfer Fcn5/1 -> Mux1/1
  Transfer Fcn4/1 -> [pT_filter], Gain - RchT (from Initialisation file)/1
  Transfer Fcn9/1 -> [pD_filter], Gain - RchD (from Initialisation file)/1
  ploss_D1/1 -> Transfer Fcn9/1, Transfer Fcn5/1, Transfer Fcn13/1, Transfer Fcn12/1, Transfer Fcn8/1, Transfer Fcn7/1, Transfer Fcn6/1
  Gain - RchT (from Initialisation file)/1 -> Sum - 1/2
  Sum of Elements/1 -> Sum - 2/2
  Sum - 1/1 -> Sum - 2/1, TcT1/1
  Sum - 2/1 -> TjT1/1
  Sum - 4/1 -> TjD1/1
  Sum - 3/1 -> Sum - 4/1, TcD1/1
  Gain - RchD (from Initialisation file)/1 -> Sum - 3/2
  Transfer Fcn10/1 -> Mux3/5
  Transfer Fcn11/1 -> Mux3/6
  Transfer Fcn12/1 -> Mux1/5
  Transfer Fcn13/1 -> Mux1/6
  [Th] -> Sum - 1/1
  [Th] -> Sum - 3/1
  [pT_filter] -> Add/1
  [pD_filter] -> Add/2
  Add/1 -> TcT2/1
  ploss_T2/1 -> Transfer Fcn4/1, Transfer Fcn11/1, Transfer Fcn10/1, Transfer Fcn3/1, Transfer Fcn2/1, Transfer Fcn1/1, Transfer Fcn/1

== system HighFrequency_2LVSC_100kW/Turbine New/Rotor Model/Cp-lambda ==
  lambda : Inport
  FromLiterature : Lookup_n-D  Commented=on  NumberOfTableDimensions=1  BreakpointsForDimension1=|  Table=|  InterpMethod=Cubic spline  InternalRulePriority=Speed  RndMeth=Simplest
      | [2.117 2.233 2.371 2.519 2.741 2.931 3.301 3.576 3.914 4.367 4.989 5.316 ...
      |             5.664 5.990 6.548 7.096 7.433 7.791 8.149 8.496 8.933 9.211 9.632 10.232 ...
      |              10.558 10.946];
      | [0.047 0.066 0.092 0.120 0.159 0.193 0.250 0.286 0.318 0.338 0.349 0.350 ...
      |             0.348 0.344 0.331 0.315 0.300 0.284 0.264 0.243 0.2115 0.190 0.154 0.093 ...
      |                 0.0584 0.0107]
  Paper_block1 : Fcn  Commented=on  Expr=(-0.0003097*u(1)^4) + (0.00952*u(1)^3) - (0.1172*u(1)^2) + (0.6269*u(1)) - 0.8487
  Saturation : Saturate  Commented=on  UpperLimit=0.393  LowerLimit=0.05
  Saturation1 : Saturate  UpperLimit=11.8  LowerLimit=0.01
  Scope : Scope
  TiPA_block : Fcn  Commented=on  Expr=(0.0011*u(1)^3) - (0.0347*u(1)^2) + (0.3178*u(1)) - 0.5032
  point_45_literature : Fcn  Commented=on  Expr=0.0195*u(1)^2*(1.3172*exp(-0.3958*u(1) + 1.539) - 0.0867*cos(0.4019*u(1) - 5.6931))
  point_45_mod_Cp : Fcn  Expr=0.000342*u(1)^4 - 0.0080558*u(1)^3 + 0.0468824*u(1)^2 - 0.0004339*u(1) + 0.045225
  Cp : Outport  VectorParamsAs1DForOutWhenUnconnected=off
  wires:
  Paper_block1/1 -> Saturation/1
  point_45_mod_Cp/1 -> Cp/1, Scope/1
  Saturation1/1 -> point_45_mod_Cp/1
  lambda/1 -> Saturation1/1

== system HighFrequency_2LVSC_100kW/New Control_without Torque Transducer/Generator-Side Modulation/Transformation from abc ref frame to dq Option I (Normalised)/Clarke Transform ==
  note: u_b
  note: u_c
  note: u_a
  note: u_alpha
  note: u_beta
  in_1 : Inport
  in_2 : Inport  Port=2
  in_3 : Inport  Port=3
  1/w2 : Constant  Value=1/sqrt(2)
  1/w6 : Constant  Value=1/sqrt(6)
  Product{,1..3} (4 alike) : Product  InputSameDT=on  RndMeth=Zero  SaturateOnIntegerOverflow=on
  Sum : Sum  Inputs=+--  InputSameDT=on  SaturateOnIntegerOverflow=on
  Sum1 : Sum  Inputs=+-  InputSameDT=on  SaturateOnIntegerOverflow=on
  w2/w3 : Constant  Value=sqrt(2/3)
  out_1 : Outport  VectorParamsAs1DForOutWhenUnconnected=off
  out_2 : Outport  Port=2  VectorParamsAs1DForOutWhenUnconnected=off
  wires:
  Product3/1 -> out_2/1
  Sum/1 -> out_1/1
  in_1/1 -> Product/2
  Product/1 -> Sum/1
  w2/w3/1 -> Product/1
  1/w6/1 -> Product1/2, Product2/2
  Product1/1 -> Sum/2
  in_2/1 -> Sum1/1, Product1/1
  in_3/1 -> Sum1/2, Product2/1
  Sum1/1 -> Product3/1
  Product2/1 -> Sum/3
  1/w2/1 -> Product3/2

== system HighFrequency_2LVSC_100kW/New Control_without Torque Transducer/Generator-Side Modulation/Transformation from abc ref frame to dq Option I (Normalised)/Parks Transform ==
  in_1 : Inport
  in_2 : Inport  Port=2
  in_3 : Inport  Port=3
  Product{,1..3} (4 alike) : Product  InputSameDT=on  RndMeth=Zero  SaturateOnIntegerOverflow=on
  Sum : Sum  Inputs=+-  InputSameDT=on  SaturateOnIntegerOverflow=on
  Sum1 : Sum  InputSameDT=on  SaturateOnIntegerOverflow=on
  cos : Fcn  Expr=cos(u(1))
  sin : Fcn  Expr=sin(u(1))
  out_1 : Outport  VectorParamsAs1DForOutWhenUnconnected=off
  out_2 : Outport  Port=2  VectorParamsAs1DForOutWhenUnconnected=off
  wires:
  Product2/1 -> Sum/2
  Product3/1 -> Sum1/1
  Product1/1 -> Sum/1
  Product/1 -> Sum1/2
  in_3/1 -> sin/1, cos/1
  sin/1 -> Product3/2, Product2/2
  cos/1 -> Product/2, Product1/2
  Sum/1 -> out_1/1
  Sum1/1 -> out_2/1
  in_1/1 -> Product3/1, Product1/1
  in_2/1 -> Product/1, Product2/1

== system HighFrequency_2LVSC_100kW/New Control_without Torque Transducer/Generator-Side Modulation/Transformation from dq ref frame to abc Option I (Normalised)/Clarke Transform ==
  in_1 : Inport
  in_2 : Inport  Port=2
  1/w2 : Constant  Value=1/sqrt(2)
  1/w6 : Constant  Value=1/sqrt(6)
  Product : Product  InputSameDT=on  RndMeth=Zero  SaturateOnIntegerOverflow=on
  Product1 : Product  InputSameDT=on  RndMeth=Zero  SaturateOnIntegerOverflow=on
  Product2 : Product  InputSameDT=on  RndMeth=Zero  SaturateOnIntegerOverflow=on
  Sum : Sum  Inputs=-+  InputSameDT=on  SaturateOnIntegerOverflow=on
  Sum1 : Sum  Inputs=--  InputSameDT=on  SaturateOnIntegerOverflow=on
  w2/w3 : Constant  Value=sqrt(2/3)
  out_1 : Outport  VectorParamsAs1DForOutWhenUnconnected=off
  out_2 : Outport  Port=2  VectorParamsAs1DForOutWhenUnconnected=off
  out_3 : Outport  Port=3  VectorParamsAs1DForOutWhenUnconnected=off
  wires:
  in_1/1 -> Product/2, Product1/1
  Product2/1 -> Sum1/2, Sum/2
  Product1/1 -> Sum1/1, Sum/1
  1/w2/1 -> Product2/2
  1/w6/1 -> Product1/2
  w2/w3/1 -> Product/1
  Product/1 -> out_1/1
  Sum/1 -> out_2/1
  in_2/1 -> Product2/1
  Sum1/1 -> out_3/1

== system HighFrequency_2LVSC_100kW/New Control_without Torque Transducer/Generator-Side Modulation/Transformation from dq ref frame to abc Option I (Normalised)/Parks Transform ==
  in_1 : Inport
  in_2 : Inport  Port=2
  in_3 : Inport  Port=3
  Product{,1..3} (4 alike) : Product  InputSameDT=on  RndMeth=Zero  SaturateOnIntegerOverflow=on
  Sum : Sum  Inputs=+-  InputSameDT=on  SaturateOnIntegerOverflow=on
  Sum1 : Sum  InputSameDT=on  SaturateOnIntegerOverflow=on
  cos : Fcn  Expr=cos(u(1))
  sin : Fcn  Expr=sin(u(1))
  out_1 : Outport  VectorParamsAs1DForOutWhenUnconnected=off
  out_2 : Outport  Port=2  VectorParamsAs1DForOutWhenUnconnected=off
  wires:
  Product2/1 -> Sum/2
  Product3/1 -> Sum1/1
  Product1/1 -> Sum/1
  Product/1 -> Sum1/2
  in_3/1 -> sin/1, cos/1
  sin/1 -> Product3/2, Product2/2
  cos/1 -> Product/2, Product1/2
  Sum/1 -> out_1/1
  Sum1/1 -> out_2/1
  in_1/1 -> Product3/1, Product1/1
  in_2/1 -> Product/1, Product2/1

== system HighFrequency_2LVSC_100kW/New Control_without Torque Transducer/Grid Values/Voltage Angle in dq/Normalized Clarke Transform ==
  a : Inport
  b : Inport  Port=2
  c : Inport  Port=3
  -1/sqrt(2) : Gain  Gain=-1/sqrt(2)
  -1/sqrt(6) : Gain  Gain=-1/sqrt(6)
  -1/sqrt(6)' : Gain  Gain=-1/sqrt(6)
  1/sqrt(2) : Gain  Gain=1/sqrt(2)
  1/sqrt(3) : Gain  Gain=1/sqrt(3)
  1/sqrt(3)' : Gain  Gain=1/sqrt(3)
  1/sqrt(3)'' : Gain  Gain=1/sqrt(3)
  Add : Sum  Inputs=+++
  Add1 : Sum
  Add2 : Sum  Inputs=+++
  sqrt(2)/sqrt(3) : Gain  Gain=sqrt(2)/sqrt(3)
  alpha : Outport  VectorParamsAs1DForOutWhenUnconnected=off
  beta : Outport  Port=2  VectorParamsAs1DForOutWhenUnconnected=off
  zero : Outport  Port=3  VectorParamsAs1DForOutWhenUnconnected=off
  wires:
  a/1 -> 1/sqrt(3)''/1, sqrt(2)/sqrt(3)/1
  sqrt(2)/sqrt(3)/1 -> Add/1
  b/1 -> 1/sqrt(3)'/1, 1/sqrt(2)/1, -1/sqrt(6)/1
  -1/sqrt(6)/1 -> Add/2
  c/1 -> 1/sqrt(3)/1, -1/sqrt(2)/1, -1/sqrt(6)'/1
  -1/sqrt(6)'/1 -> Add/3
  Add/1 -> alpha/1
  Add1/1 -> beta/1
  1/sqrt(2)/1 -> Add1/1
  -1/sqrt(2)/1 -> Add1/2
  1/sqrt(3)/1 -> Add2/3
  1/sqrt(3)'/1 -> Add2/2
  1/sqrt(3)''/1 -> Add2/1
  Add2/1 -> zero/1

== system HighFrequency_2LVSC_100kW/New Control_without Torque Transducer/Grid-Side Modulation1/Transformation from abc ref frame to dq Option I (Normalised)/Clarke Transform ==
  note: u_b
  note: u_c
  note: u_a
  note: u_alpha
  note: u_beta
  in_1 : Inport
  in_2 : Inport  Port=2
  in_3 : Inport  Port=3
  1/w2 : Constant  Value=1/sqrt(2)
  1/w6 : Constant  Value=1/sqrt(6)
  Product{,1..3} (4 alike) : Product  InputSameDT=on  RndMeth=Zero  SaturateOnIntegerOverflow=on
  Sum : Sum  Inputs=+--  InputSameDT=on  SaturateOnIntegerOverflow=on
  Sum1 : Sum  Inputs=+-  InputSameDT=on  SaturateOnIntegerOverflow=on
  w2/w3 : Constant  Value=sqrt(2/3)
  out_1 : Outport  VectorParamsAs1DForOutWhenUnconnected=off
  out_2 : Outport  Port=2  VectorParamsAs1DForOutWhenUnconnected=off
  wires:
  Product3/1 -> out_2/1
  Sum/1 -> out_1/1
  in_1/1 -> Product/2
  Product/1 -> Sum/1
  w2/w3/1 -> Product/1
  1/w6/1 -> Product1/2, Product2/2
  Product1/1 -> Sum/2
  in_2/1 -> Sum1/1, Product1/1
  in_3/1 -> Sum1/2, Product2/1
  Sum1/1 -> Product3/1
  Product2/1 -> Sum/3
  1/w2/1 -> Product3/2

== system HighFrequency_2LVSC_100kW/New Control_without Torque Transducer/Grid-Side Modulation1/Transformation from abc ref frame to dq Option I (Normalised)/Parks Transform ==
  in_1 : Inport
  in_2 : Inport  Port=2
  in_3 : Inport  Port=3
  Product{,1..3} (4 alike) : Product  InputSameDT=on  RndMeth=Zero  SaturateOnIntegerOverflow=on
  Sum : Sum  Inputs=+-  InputSameDT=on  SaturateOnIntegerOverflow=on
  Sum1 : Sum  InputSameDT=on  SaturateOnIntegerOverflow=on
  cos : Fcn  Expr=cos(u(1))
  sin : Fcn  Expr=sin(u(1))
  out_1 : Outport  VectorParamsAs1DForOutWhenUnconnected=off
  out_2 : Outport  Port=2  VectorParamsAs1DForOutWhenUnconnected=off
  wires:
  Product2/1 -> Sum/2
  Product3/1 -> Sum1/1
  Product1/1 -> Sum/1
  Product/1 -> Sum1/2
  in_3/1 -> sin/1, cos/1
  sin/1 -> Product3/2, Product2/2
  cos/1 -> Product/2, Product1/2
  Sum/1 -> out_1/1
  Sum1/1 -> out_2/1
  in_1/1 -> Product3/1, Product1/1
  in_2/1 -> Product/1, Product2/1

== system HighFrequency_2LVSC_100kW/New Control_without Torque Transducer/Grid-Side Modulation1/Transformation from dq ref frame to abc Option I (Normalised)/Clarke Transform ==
  in_1 : Inport
  in_2 : Inport  Port=2
  1/w2 : Constant  Value=1/sqrt(2)
  1/w6 : Constant  Value=1/sqrt(6)
  Product : Product  InputSameDT=on  RndMeth=Zero  SaturateOnIntegerOverflow=on
  Product1 : Product  InputSameDT=on  RndMeth=Zero  SaturateOnIntegerOverflow=on
  Product2 : Product  InputSameDT=on  RndMeth=Zero  SaturateOnIntegerOverflow=on
  Sum : Sum  Inputs=-+  InputSameDT=on  SaturateOnIntegerOverflow=on
  Sum1 : Sum  Inputs=--  InputSameDT=on  SaturateOnIntegerOverflow=on
  w2/w3 : Constant  Value=sqrt(2/3)
  out_1 : Outport  VectorParamsAs1DForOutWhenUnconnected=off
  out_2 : Outport  Port=2  VectorParamsAs1DForOutWhenUnconnected=off
  out_3 : Outport  Port=3  VectorParamsAs1DForOutWhenUnconnected=off
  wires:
  in_1/1 -> Product/2, Product1/1
  Product2/1 -> Sum1/2, Sum/2
  Product1/1 -> Sum1/1, Sum/1
  1/w2/1 -> Product2/2
  1/w6/1 -> Product1/2
  w2/w3/1 -> Product/1
  Product/1 -> out_1/1
  Sum/1 -> out_2/1
  in_2/1 -> Product2/1
  Sum1/1 -> out_3/1

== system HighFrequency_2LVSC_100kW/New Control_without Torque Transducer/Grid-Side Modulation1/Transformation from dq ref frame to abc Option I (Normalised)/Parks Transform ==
  in_1 : Inport
  in_2 : Inport  Port=2
  in_3 : Inport  Port=3
  Product{,1..3} (4 alike) : Product  InputSameDT=on  RndMeth=Zero  SaturateOnIntegerOverflow=on
  Sum : Sum  Inputs=+-  InputSameDT=on  SaturateOnIntegerOverflow=on
  Sum1 : Sum  InputSameDT=on  SaturateOnIntegerOverflow=on
  cos : Fcn  Expr=cos(u(1))
  sin : Fcn  Expr=sin(u(1))
  out_1 : Outport  VectorParamsAs1DForOutWhenUnconnected=off
  out_2 : Outport  Port=2  VectorParamsAs1DForOutWhenUnconnected=off
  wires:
  Product2/1 -> Sum/2
  Product3/1 -> Sum1/1
  Product1/1 -> Sum/1
  Product/1 -> Sum1/2
  in_3/1 -> sin/1, cos/1
  sin/1 -> Product3/2, Product2/2
  cos/1 -> Product/2, Product1/2
  Sum/1 -> out_1/1
  Sum1/1 -> out_2/1
  in_1/1 -> Product3/1, Product1/1
  in_2/1 -> Product/1, Product2/1

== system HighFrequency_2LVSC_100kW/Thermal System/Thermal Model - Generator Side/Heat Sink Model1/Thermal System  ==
  P1/D1 : Inport
  1/R_th : Inport  Port=2
  C : Inport  Port=3
  Add : Sum  Inputs=+-
  Integrator : Integrator
  Math Function1 : Math  Operator=reciprocal  SignedPower=on
  Product : Product
  Product1 : Product
  Tha : Outport  VectorParamsAs1DForOutWhenUnconnected=off
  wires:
  Integrator/1 -> Product/2, Tha/1
  C/1 -> Math Function1/1
  P1/D1/1 -> Add/1
  1/R_th/1 -> Product/1
  Product/1 -> Add/2
  Add/1 -> Product1/2
  Math Function1/1 -> Product1/1
  Product1/1 -> Integrator/1

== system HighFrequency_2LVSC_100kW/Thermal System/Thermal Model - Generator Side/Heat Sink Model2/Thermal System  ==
  P1/D1 : Inport
  1/R_th : Inport  Port=2
  C : Inport  Port=3
  Add : Sum  Inputs=+-
  Integrator : Integrator
  Math Function1 : Math  Operator=reciprocal  SignedPower=on
  Product : Product
  Product1 : Product
  Tha : Outport  VectorParamsAs1DForOutWhenUnconnected=off
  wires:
  Integrator/1 -> Product/2, Tha/1
  C/1 -> Math Function1/1
  P1/D1/1 -> Add/1
  1/R_th/1 -> Product/1
  Product/1 -> Add/2
  Add/1 -> Product1/2
  Math Function1/1 -> Product1/1
  Product1/1 -> Integrator/1

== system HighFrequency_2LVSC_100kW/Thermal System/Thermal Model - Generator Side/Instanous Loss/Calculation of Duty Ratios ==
  Dabc : Inport
  Bias - 1 : Constant
  Sum - 1 : Sum  Inputs=+-
  D_T1 : Outport  VectorParamsAs1DForOutWhenUnconnected=off
  D_D1 : Outport  Port=2  VectorParamsAs1DForOutWhenUnconnected=off
  D_T2 : Outport  Port=3  VectorParamsAs1DForOutWhenUnconnected=off
  D_D2 : Outport  Port=4  VectorParamsAs1DForOutWhenUnconnected=off
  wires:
  Bias - 1/1 -> Sum - 1/1
  Dabc/1 -> Sum - 1/2, D_D1/1, D_T1/1
  Sum - 1/1 -> D_D2/1, D_T2/1
